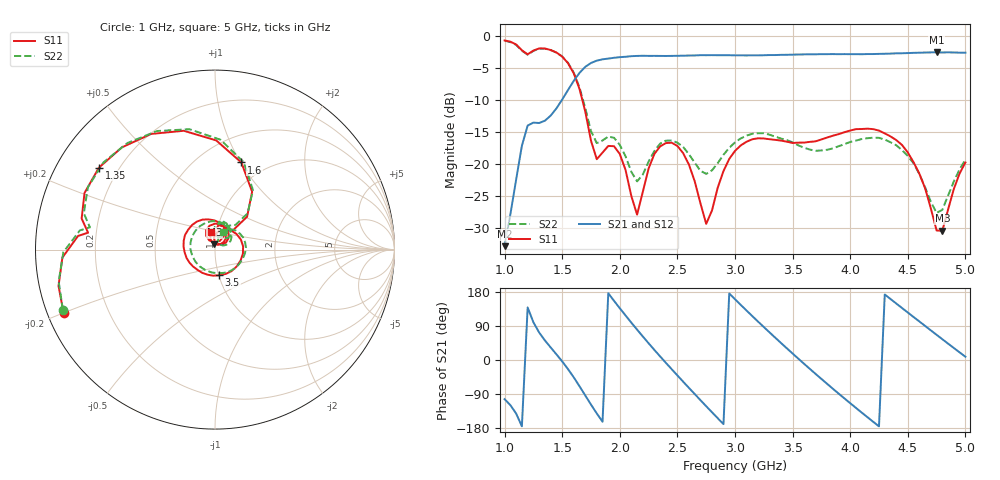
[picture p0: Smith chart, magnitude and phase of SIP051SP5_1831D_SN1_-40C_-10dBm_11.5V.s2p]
# GHz  S  dB  R  50
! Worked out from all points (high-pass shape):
!   81 points, 1 GHz to 5 GHz, reference 50 ohm
!   highest |S21| = -2.63 dB at 4.75 GHz (marker M1); lowest = -32.9 dB at 1 GHz (marker M2)
!   |S21| within 3 dB of the highest: 1.661 GHz to end of sweep
!   lowest |S11| = -30.5 dB at 4.8 GHz (marker M3), VSWR 1.06, Z = 49.5 + j2.94 ohm
!   |S11| at or under -10 dB: 1.674 GHz to end of sweep
!   |S22| runs from -27.7 to -0.8 dB; largest |S21 - S12| = 0.003
!   S11 on the Smith chart (normalised r, x): 1 GHz: 0.05, -0.20; 1.35 GHz: 0.13, +0.31; 1.6 GHz: 0.77, +1.01; 3.5 GHz: 1.01, -0.29; 5 GHz: 0.94, +0.19
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1  -0.77 -157.2  -32.90 -103.3  -32.99 -103.7  -0.80 -158.4
1.2  -2.94 172.4  -14.06 138.7  -14.04 138.7  -3.00 169.9
1.35  -2.03 144.7  -13.30 51.6  -13.28 51.6  -2.06 142.0
1.5  -3.29 104.7  -10.00 -3.7  -9.97 -3.8  -3.28 101.9
1.6  -5.90 73.2  -7.09 -45.7  -7.09 -45.8  -5.80 71.8
1.7  -11.86 45.7  -4.89 -93.5  -4.89 -93.5  -11.32 48.0
1.8  -19.32 70.4  -3.93 -140.9  -3.93 -140.9  -16.80 65.4
1.95  -17.29 73.4  -3.48 156.0  -3.48 156.1  -15.97 65.6
2.15  -27.98 95.3  -3.19 80.2  -3.19 80.2  -22.78 72.8
2.35  -17.31 102.9  -3.19 9.4  -3.19 9.5  -16.88 83.6
2.65  -22.74 32.7  -3.12 -89.7  -3.10 -89.8  -19.85 41.8
2.75  -29.41 61.9  -3.08 -122.0  -3.07 -122.0  -21.61 53.5
3  -18.02 64.1  -3.10 160.3  -3.09 160.4  -16.69 50.4
3.25  -16.08 -7.9  -3.08 87.1  -3.08 87.0  -15.26 3.1
3.5  -16.78 -80.7  -2.99 17.1  -2.99 17.1  -16.69 -55.6
3.7  -16.52 -130.8  -2.93 -36.8  -2.93 -36.8  -18.00 -115.9
4  -14.84 164.5  -2.92 -113.9  -2.91 -113.9  -16.62 149.6
4.35  -15.76 91.3  -2.82 161.0  -2.84 161.0  -16.67 65.5
4.55  -19.78 53.5  -2.71 113.5  -2.71 113.5  -19.96 29.8
4.75  -30.45 65.2  -2.63 66.4  -2.65 66.5  -27.70 40.8
4.8  -30.49 97.2  -2.65 54.8  -2.64 54.8  -27.22 60.9
5  -19.83 101.7  -2.69 8.7  -2.70 8.6  -19.37 66.8
